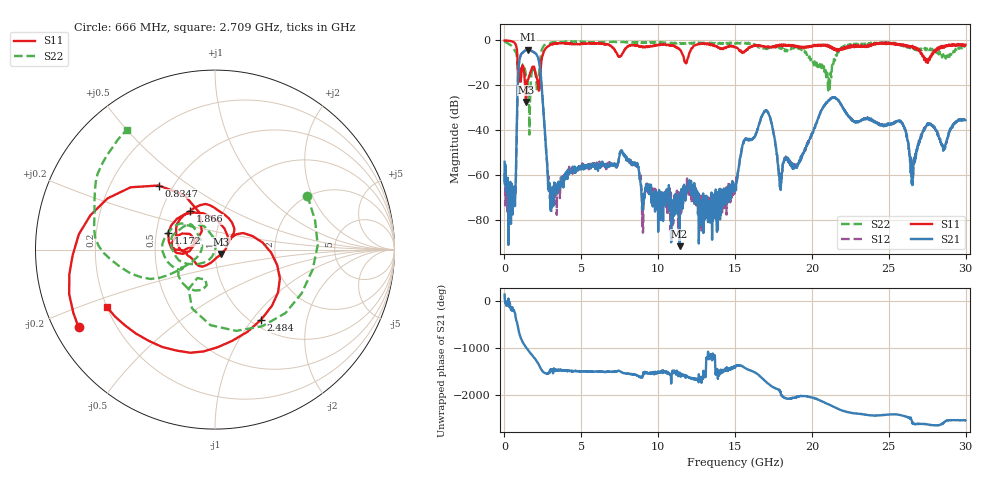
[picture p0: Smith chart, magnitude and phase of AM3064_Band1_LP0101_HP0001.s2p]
# Hz S DB R 50.0
!freq dBS11 angS11 dBS21 angS21 dBS12 angS12 dBS22 angS22
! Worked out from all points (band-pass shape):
!   1600 points, 10 MHz to 29.98 GHz, reference 50 ohm
!   highest |S21| = -4.16 dB at 1.528 GHz (marker M1); lowest = -91.5 dB at 11.39 GHz (marker M2)
!   |S21| within 3 dB of the highest: 1.029 GHz to 2.155 GHz (1.126 GHz wide, 70.7 % of centre)
!   lowest |S11| = -27.4 dB at 1.397 GHz (marker M3), VSWR 1.09, Z = 53.6 - j2.57 ohm
!   |S11| at or under -10 dB: 857.5 MHz to 2.391 GHz (1.534 GHz wide, 94.4 % of centre); 11.78358 GHz to 11.8396 GHz (56.02 MHz wide, 0.474 % of centre); 27.52547 GHz to 27.52934 GHz (3.868 MHz wide, 0.014 % of centre)
!   |S22| runs from -41.9 to -0.4 dB; largest |S21 - S12| = 0.0084
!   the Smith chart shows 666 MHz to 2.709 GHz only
!   S11 on the Smith chart (normalised r, x): 666 MHz: 0.07, -0.26; 834.7 MHz: 0.42, +0.39; 1.172 GHz: 0.58, +0.12; 1.866 GHz: 0.70, +0.32; 2.484 GHz: 1.11, -1.11; 2.709 GHz: 0.20, -0.24
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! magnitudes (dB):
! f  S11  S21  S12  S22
! 10 MHz  -0.1  -54.0  -58.8  -0.4
! 666 MHz  -1.2  -67.7  -64.6  -4.5
! 834.7 MHz  -6.5  -27.4  -27.4  -9.1
! 1.172 GHz  -11.2  -5.5  -5.5  -10.9
! 1.397 GHz  -27.4  -4.3  -4.3  -15.4
! 1.528 GHz  -17.5  -4.2  -4.1  -19.0
! 1.866 GHz  -11.8  -5.1  -5.1  -12.1
! 2.484 GHz  -6.6  -26.2  -26.2  -3.3
! 2.709 GHz  -3.3  -47.6  -48.3  -1.6
! 3.046 GHz  -1.8  -73.0  -76.4  -1.0
! 5.015 GHz  -1.4  -56.4  -56.5  -0.8
! 7.657 GHz  -5.9  -49.3  -49.6  -0.7
! 10 GHz  -2.0  -85.1  -72.2  -1.0
! 11.39 GHz  -4.0  -91.5  -69.0  -1.3
! 15 GHz  -2.9  -65.5  -63.9  -1.4
! 16.94 GHz  -2.7  -31.6  -31.4  -3.6
! 17.93 GHz  -2.1  -64.1  -64.8  -2.9
! 19.99 GHz  -2.8  -41.8  -41.9  -9.4
! 21.4 GHz  -3.4  -25.5  -25.4  -10.5
! 25 GHz  -1.0  -37.4  -37.4  -1.2
! 26.53 GHz  -2.4  -64.4  -56.6  -4.3
! 29.98 GHz  -1.9  -35.5  -35.2  -2.9
